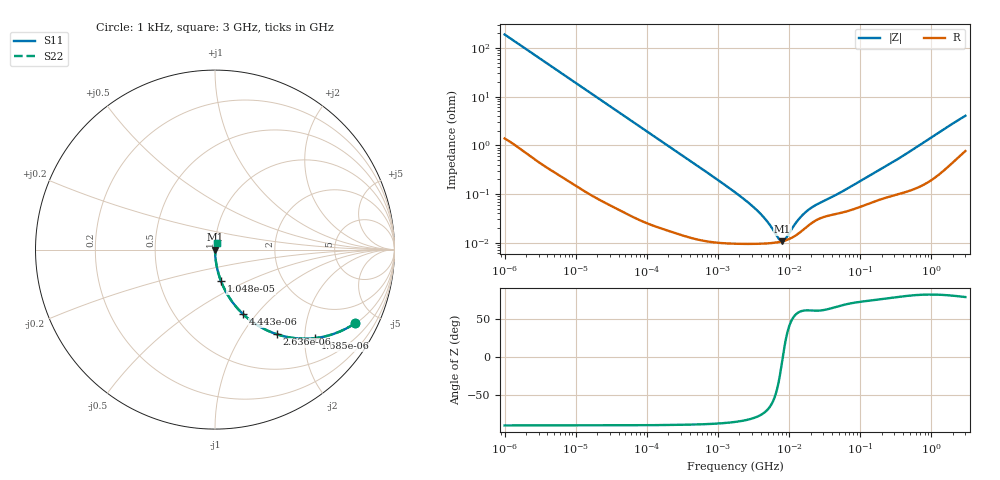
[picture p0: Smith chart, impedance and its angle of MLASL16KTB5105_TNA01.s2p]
! MLASL16KTB5105_TNA01  S-PARAMETER MODEL  ( Standard Model )
! Model Generated by TAIYO YUDEN Corporation (http://www.ty-top.com)
! Version 1.0
! TAIYO YUDEN Control No. 220601
! Copyright(c) 2008 TAIYO YUDEN CO.,LTD. All Rights Reserved.
! Product Description (link to TY-COMPAS)
! https://ds.yuden.co.jp/TYCOMPAS/or/detail?pn=MLASL16KTB5105KTNA01&u=M
! Products Name : Multilayer Ceramic Capacitors
! Characteristics :
!  Capacitance : 1 [uF] , Rated Voltage : 10 [V] , TCC : X5R
!  Case Size : 1.6 x 0.8 / 0.063 x 0.031 [mm/inch] , Thickness : 0.45 / 0.018 [mm/inch]
!  (Conditions: Temperature = 25 [degC] , DC Bias Voltage = 0 [V])
! External Node Assignments :
!  1  o---| |---o  2
! GND o---------o GND
! Frequency Range : 1kHz  -  3GHz  [ 401 STEP ]
# MHZ S RI R 50
! Freq[MHz].  S11 Real  S11 Imag  S21 Real  S21 Imag  S12 Real  S12 Imag  S22 Real  S22 Imag
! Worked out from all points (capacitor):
!   401 points, 1 kHz to 3 GHz, reference 50 ohm
!   read as one part in series: C = 840 nF near 1.077 kHz
!   lowest |Z| = 10.7 mohm at 7.989 MHz (marker M1)
!   series resonance near 8.135 MHz, so ESL is about 460 pH
!   S11 on the Smith chart (normalised r, x): 1 kHz: 1.03, -3.78; 1.685 kHz: 1.02, -2.25; 2.636 kHz: 1.01, -1.44; 4.443 kHz: 1.01, -0.86; 10.47 kHz: 1.00, -0.37; 3 GHz: 1.02, +0.08
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0.001  0.7798 -0.4107  0.2202 0.4107  0.2202 0.4107  0.7798 -0.4107
0.001685  0.5584 -0.4929  0.4416 0.4929  0.4416 0.4929  0.5584 -0.4929
0.002636  0.3431 -0.4712  0.6569 0.4712  0.6569 0.4712  0.3431 -0.4712
0.004443  0.1571 -0.3602  0.8429 0.3602  0.8429 0.3602  0.1571 -0.3602
0.006451  0.0821 -0.2709  0.9179 0.2709  0.9179 0.2709  0.0821 -0.2709
0.010475  0.0335 -0.1762  0.9665 0.1762  0.9665 0.1762  0.0335 -0.1762
0.01216  0.0253 -0.1532  0.9747 0.1532  0.9747 0.1532  0.0253 -0.1532
0.033275  0.00387 -0.0575  0.9961 0.0575  0.9961 0.0575  0.00387 -0.0575
0.147855  0.000374 -0.0131  0.9996 0.0131  0.9996 0.0131  0.000374 -0.0131
1.732051  9.62e-05 -0.00108  0.9999 0.00108  0.9999 0.00108  9.62e-05 -0.00108
2.812335  9.46e-05 -0.000615  0.9999 0.000615  0.9999 0.000615  9.46e-05 -0.000615
3.93371  9.52e-05 -0.000384  0.9999 0.000384  0.9999 0.000384  9.52e-05 -0.000384
5.106836  9.7e-05 -0.000234  0.9999 0.000234  0.9999 0.000234  9.7e-05 -0.000234
7.143107  0.000103 -6.37e-05  0.9999 6.37e-05  0.9999 6.37e-05  0.000103 -6.37e-05
7.988506  0.000107 -8.8e-06  0.9999 8.8e-06  0.9999 8.8e-06  0.000107 -8.8e-06
8.933959  0.000112 4.61e-05  0.9999 -4.61e-05  0.9999 -4.61e-05  0.000112 4.61e-05
12.03889  0.000137 0.000196  0.9999 -0.000196  0.9999 -0.000196  0.000137 0.000196
14.50609  0.000167 0.000292  0.9998 -0.000292  0.9998 -0.000292  0.000167 0.000292
21.06097  0.000257 0.00047  0.9997 -0.00047  0.9997 -0.00047  0.000257 0.00047
55.52535  0.000416 0.00104  0.9996 -0.00104  0.9996 -0.00104  0.000416 0.00104
256.0921  0.000895 0.00399  0.9991 -0.00399  0.9991 -0.00399  0.000895 0.00399
3000  0.00911 0.039  0.9909 -0.039  0.9909 -0.039  0.00911 0.039
